TYPE "ST_ConnectionSettings"
VERSION : 0.1


  STRUCT
   tTimeout : TIME  := T#2S;	//Timeout | Timeout of the connection | Unit [ms]
   stProfinet : "ST_ProfinetIO";	//This structure contains all da required for a connection via PROFINET
  END_STRUCT ;
END_TYPE

